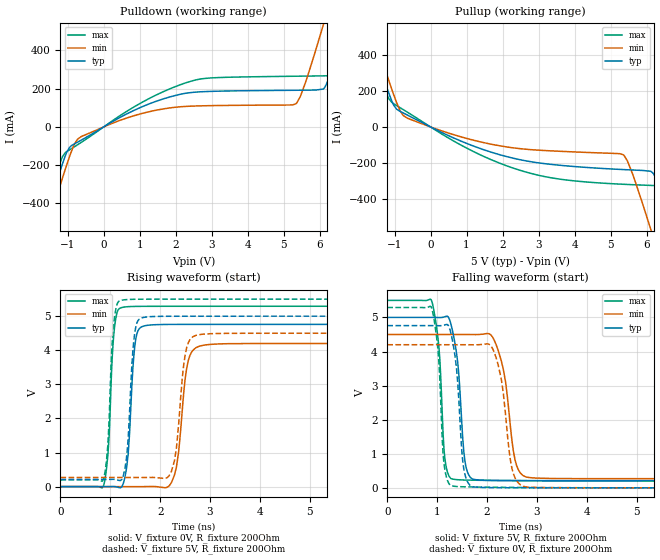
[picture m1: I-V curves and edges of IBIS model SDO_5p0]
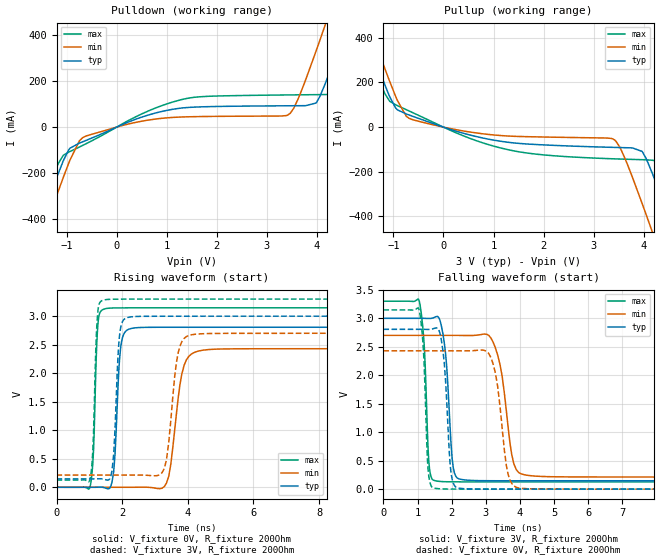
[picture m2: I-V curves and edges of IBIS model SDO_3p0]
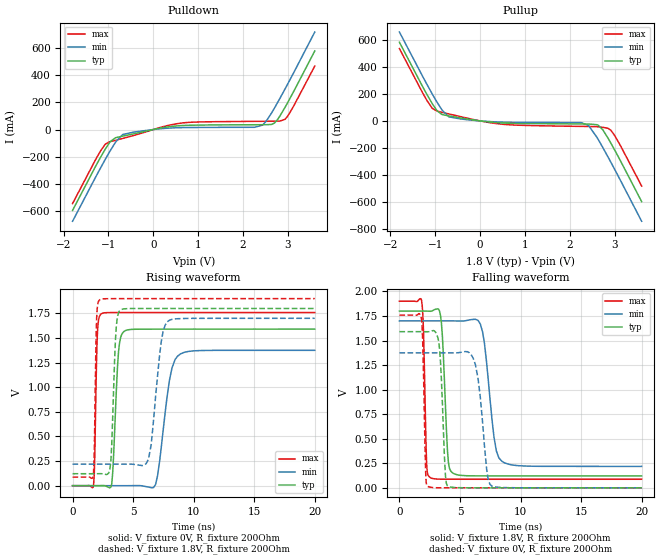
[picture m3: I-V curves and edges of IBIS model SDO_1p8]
|Texas Instruments Incorporated
|Quad, True 14-Bit, SPI Voltage-Output DAC With Precision Internal Reference
[IBIS Ver]   4.1
[File name]   dacx0504.ibs
[File Rev]   1.0
[Date]   01/27/2017
[Source]
| Texas Instruments Incorporated.
| 12500 TI Blvd
| Dallas, TX -75243
[Notes]   Revision History:
| Rev 1.0: 01/27/2017
| - Initial version of the model
| - Model generated from simulations in TISPICE
| - C_comp although listed in numerical order of value are
|   obtained from varying PVT conditions. For PVT conditions for
|   each specific value refer the buffer description under
|   respective [Model]. IBIS model user is responsible for using
|   appropriate C_comp to simulate for Signal Integrity.
| - Warnings regarding combined Non-monotonicity of various models have been
|   reviewd and considered minor and can be ignored.
| - Model names with a trailing _1p8 contain the model for
|   1.8V operation. Model names with a trailing _3p0 contain the model
|   for 3.3V operation.Model names with a trailing _5p0 contain the model
|   for 5.0V operation.
[Disclaimer]
| This model is designed as an aid for customers of Texas Instruments.
| TI and its licensors and suppliers make no warranties, either expressed
| or implied, with respect to this  model, including the warranties of
| merchantability or fitness for a particular purpose. The model is
| provided solely on an "as is" basis. The entire risk as to its quality
| and performance is with the customer.
[Copyright]
 (C) Copyright 2017 Texas Instruments Incorporated.All rights reserved.
|   Device
[Component]  DAC70504RTE
[Manufacturer]   TI
[Package]  |16 pin WQFN
| variable   typ   min   max
R_pkg   0.1   0.08   0.12
L_pkg   1.0nH   0.8nH   1.2nH
C_pkg   0.2pF   0.16pF   0.24pF
[Pin]   signal_name   model_name   R_pin   L_pin   C_pin
1   REF   NC   NA   NA   NA
2   OUT0   NC   NA   NA   NA
3   OUT1   NC   NA   NA   NA
4   OUT2   NC   NA   NA   NA
5   OUT3   NC   NA   NA   NA
6   GND   GND   NA   NA   NA
7   VDD   POWER   NA   NA   NA
8   GAIN   SDI   NA   NA   NA
9   RSTSEL   SDI   NA   NA   NA
10   REFDIV   SDI   NA   NA   NA
11   LDACB   SDI   NA   NA   NA
12   CSB   SDI   NA   NA   NA
13   SCLK   SDI   NA   NA   NA
14   SDI   SDI   NA   NA   NA
15   SDO/ALARMB   SDO   NA   NA   NA
16   VIO   POWER   NA   NA   NA
|   Model Selectors
[Model Selector]  SDO
SDO_5p0  sdata buffer at 5.0V operation.
SDO_3p0  sdata buffer at 3.0V operation.
SDO_1p8  sdata buffer at 1.8V operation.
[Model Selector]  SDI
SDI_5p0  sdata buffer at 5.0V operation.
SDI_3p0  sdata buffer at 3.0V operation.
SDI_1p8  sdata buffer at 1.8V operation.
| Models and submodels in the file (6): SDO_5p0 (Output), SDO_3p0 (Output), SDO_1p8 (Output), SDI_5p0 (Input), SDI_3p0 (Input), SDI_1p8 (Input)
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|   Model
[Model]   SDO_5p0
Model_type   Output
Polarity   Non-Inverting
Vmeas = 2.5
Vref = 0
Cref = 1pF
Rref = 100000
|   typ   min   max
C_comp   1pF   1pF   1pF
[Voltage Range]   5   4.5   5.5
[Temperature Range]   27   125   -40
[Pullup Reference]   5   4.5   5.5
[Pulldown Reference]   0   0   0
[Power Clamp Reference]   5   4.5   5.5
[GND Clamp Reference]   0   0   0
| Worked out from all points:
|   slope of the pulldown table from 0 to 0.75 V, typ, clamps not added: 9.61 ohm
|   slope of the pullup table from 0 to 0.75 V, typ, clamps not added: 10.7 ohm
|   falling waveform, V_fixture 5V, R_fixture 200Ohm: 20-80 % time 149ps typ, 227ps min, 119ps max; typ from 5 V to 0.211 V
|   rising waveform, V_fixture 0V, R_fixture 200Ohm: 20-80 % time 112ps typ, 167ps min, 100ps max; typ from 0 V to 4.76 V
|   rising waveform, V_fixture 5V, R_fixture 200Ohm: 20-80 % time 111ps typ, 156ps min, 96.4ps max; typ from 0.211 V to 5 V
|   falling waveform, V_fixture 0V, R_fixture 200Ohm: 20-80 % time 139ps typ, 206ps min, 114ps max; typ from 4.76 V to 0 V
[Pulldown]
|   Voltage   I(typ)   I(min)   I(max)
-5V       -2.704A    -2.779A    -2.658A
-2.195V   -855.7mA   -935.1mA   -805.9mA
-1.58V    -458.8mA   -539.1mA   -408.2mA
-1.145V   -193.2mA   -268.4mA   -155.8mA
-725mV    -79.65mA   -64.21mA   -93.36mA
640mV     67.98mA    46.69mA    81.52mA
2.65V     183.4mA    110.1mA    249.6mA
5.335V    191.9mA    120.8mA    265.3mA
6.1V      198.3mA    533.1mA    267.3mA
6.805V    589.9mA    986.3mA    275.3mA
7.27V     890.2mA    1.289A     522.8mA
10V       2.688A     3.088A     2.314A
[Pullup]
|   Voltage   I(typ)   I(min)   I(max)
-5V       2.688A     2.757A     2.645A
-2.15V    810.1mA    884.5mA    764mA
-1.73V    538.5mA    613.7mA    491.9mA
-1.655V   490.6mA    565.7mA    443.9mA
-1.16V    187.2mA    257.5mA    156mA
-755mV    76.9mA     62.84mA    95.4mA
2.245V    -170.6mA   -114.3mA   -224.3mA
5.35V     -235.8mA   -153.8mA   -317.2mA
6.1V      -245mA     -555.8mA   -323.4mA
6.865V    -646.4mA   -1.048A    -338.7mA
7.3V      -927.2mA   -1.331A    -557.5mA
10V       -2.705A    -3.11A     -2.328A
[Ramp]
R_load = 200
|   typ   min   max
dV/dt_r   2.85629/1.11775e-10   2.51978/1.67498e-10   3.17481/1.00389e-10
dV/dt_f   2.87354/1.49374e-10   2.53929/2.27194e-10   3.18142/1.19398e-10
[Falling Waveform]
V_fixture = 5V
V_fixture_min = 4.5V
V_fixture_max = 5.5V
R_fixture = 200Ohm
C_fixture = 0F
|   Time   V(typ)   V(min)   V(max)
0s        5V         4.5V       5.5V
880.1ps   5V         4.5V       5.521V
1.037ns   4.997V     4.5V       4.086V
1.153ns   5.02V      4.5V       881.8mV
1.317ns   4.547V     4.5V       255.7mV
1.555ns   801.4mV    4.5V       229.4mV
1.767ns   241.5mV    4.497V     224.1mV
2.181ns   217mV      4.205V     215.8mV
2.852ns   213.6mV    301.8mV    207.9mV
20ns      210.7mV    267.8mV    197.6mV
[Rising Waveform]
V_fixture = 0V
V_fixture_min = 0V
V_fixture_max = 0V
R_fixture = 200Ohm
C_fixture = 0F
|   Time   V(typ)   V(min)   V(max)
0s        19.62uV    26.57uV    14.41uV
861.1ps   -180.9uV   -40.74uV   7.327mV
1.087ns   861.4uV    -58.37uV   4.697V
1.275ns   167.7mV    -73.07uV   5.267V
1.511ns   4.328V     -91.53uV   5.286V
1.712ns   4.724V     1.13mV     5.288V
2.225ns   4.758V     113.5mV    5.291V
2.562ns   4.759V     3.688V     5.291V
2.929ns   4.759V     4.16V      5.291V
20ns      4.761V     4.2V       5.291V
[Rising Waveform]
V_fixture = 5V
V_fixture_min = 4.5V
V_fixture_max = 5.5V
R_fixture = 200Ohm
C_fixture = 0F
|   Time   V(typ)   V(min)   V(max)
0s        210.7mV    267.8mV    197.6mV
861.1ps   210.6mV    267.8mV    206.8mV
1.069ns   213.7mV    267.8mV    4.778V
1.236ns   229.2mV    267.8mV    5.471V
1.49ns    4.509V     267.8mV    5.496V
1.666ns   4.963V     268mV      5.498V
2.225ns   4.997V     442.6mV    5.499V
2.502ns   4.999V     3.87V      5.499V
2.783ns   4.999V     4.458V     5.499V
20ns      5V         4.5V       5.5V
[Falling Waveform]
|Gnd
V_fixture = 0V
V_fixture_min = 0V
V_fixture_max = 0V
R_fixture = 200Ohm
C_fixture = 0F
|   Time   V(typ)   V(min)   V(max)
0s        4.761V     4.2V       5.291V
880.1ps   4.761V     4.2V       5.311V
1.137ns   4.775V     4.2V       709.1mV
1.317ns   4.241V     4.2V       52.06mV
1.533ns   562.4mV    4.2V       31.34mV
1.712ns   31.19mV    4.198V     25.67mV
2.143ns   5.842mV    3.982V     17.63mV
2.502ns   2.991mV    560mV      13.5mV
2.783ns   2.259mV    25.26mV    10.82mV
20ns      19.87uV    27.03uV    14.9uV
|   Model
[Model]   SDO_3p0
Model_type   Output
Polarity   Non-Inverting
Vmeas = 1.5
Vref = 0
Cref = 1pF
Rref = 100000
|   typ   min   max
C_comp   1pF   1pF   1pF
[Voltage Range]   3   2.7   3.3
[Temperature Range]   27   125   -40
[Pullup Reference]   3   2.7   3.3
[Pulldown Reference]   0   0   0
[Power Clamp Reference]   3   2.7   3.3
[GND Clamp Reference]   0   0   0
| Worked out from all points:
|   slope of the pulldown table from 0 to 0.45 V, typ, clamps not added: 11.3 ohm
|   slope of the pullup table from 0 to 0.45 V, typ, clamps not added: 14.7 ohm
|   falling waveform, V_fixture 3V, R_fixture 200Ohm: 20-80 % time 179ps typ, 323ps min, 126ps max; typ from 3 V to 0.147 V
|   rising waveform, V_fixture 0V, R_fixture 200Ohm: 20-80 % time 141ps typ, 306ps min, 101ps max; typ from 0 V to 2.81 V
|   rising waveform, V_fixture 3V, R_fixture 200Ohm: 20-80 % time 133ps typ, 256ps min, 99.8ps max; typ from 0.147 V to 3 V
|   falling waveform, V_fixture 0V, R_fixture 200Ohm: 20-80 % time 162ps typ, 279ps min, 119ps max; typ from 2.81 V to 0 V
[Pulldown]
|   Voltage   I(typ)   I(min)   I(max)
-3V       -1.383A    -1.461A    -1.334A
-1.74V    -560.3mA   -640.6mA   -509.8mA
-1.29V    -276.3mA   -355.7mA   -227.6mA
-1.065V   -146.5mA   -219.1mA   -122.6mA
-606mV    -57.46mA   -38.41mA   -71.8mA
1.329V    83.93mA    44.43mA    121.6mA
3.417V    93.05mA    52.27mA    140.3mA
3.984V    105.1mA    331.4mA    141.5mA
4.173V    192.7mA    449.4mA    142mA
4.65V     486.8mA    754.4mA    254mA
4.902V    648.8mA    917.7mA    410mA
6V        1.366A     1.636A     1.124A
[Pullup]
|   Voltage   I(typ)   I(min)   I(max)
-3V       1.366A     1.439A     1.322A
-1.749V   549.7mA    625mA      503mA
-1.074V   136mA      204.5mA    115.8mA
-615mV    48.56mA    33.25mA    64.91mA
1.275V    -67.36mA   -39.59mA   -100.3mA
3.381V    -90.56mA   -52.6mA    -141.7mA
3.966V    -108.5mA   -340.8mA   -145.8mA
4.173V    -207.5mA   -470.3mA   -148.4mA
4.506V    -411.3mA   -683mA     -188.9mA
4.767V    -577.9mA   -851.6mA   -338.2mA
4.893V    -659.2mA   -933.3mA   -417.3mA
6V        -1.383A    -1.658A    -1.137A
[Ramp]
R_load = 200
|   typ   min   max
dV/dt_r   1.68391/1.41258e-10   1.45763/3.05913e-10   1.88848/1.00573e-10
dV/dt_f   1.71187/1.78517e-10   1.49191/3.23449e-10   1.90378/1.2617e-10
[Falling Waveform]
V_fixture = 3V
V_fixture_min = 2.7V
V_fixture_max = 3.3V
R_fixture = 200Ohm
C_fixture = 0F
|   Time   V(typ)   V(min)   V(max)
0s        3V         2.7V       3.3V
1.05ns    3V         2.7V       3.307V
1.192ns   2.999V     2.7V       2.559V
1.328ns   2.997V     2.7V       501.8mV
1.526ns   3.025V     2.7V       147.3mV
2.046ns   381.1mV    2.7V       129.5mV
2.257ns   174.5mV    2.699V     128.4mV
3.213ns   148mV      2.583V     127.7mV
4.12ns    147.6mV    254.1mV    127.6mV
20ns      146.9mV    213.5mV    127mV
[Rising Waveform]
V_fixture = 0V
V_fixture_min = 0V
V_fixture_max = 0V
R_fixture = 200Ohm
C_fixture = 0F
|   Time   V(typ)   V(min)   V(max)
0s        14.5uV     22.32uV    10.14uV
1.025ns   -63.32uV   -17.54uV   13.71mV
1.266ns   1.454mV    -26.94uV   2.893V
1.461ns   -8.28mV    -34.49uV   3.127V
1.985ns   2.561V     -54.88uV   3.145V
2.257ns   2.781V     -65.46uV   3.146V
3.347ns   2.806V     68.51mV    3.147V
3.82ns    2.806V     1.988V     3.147V
4.316ns   2.806V     2.387V     3.147V
20ns      2.807V     2.429V     3.147V
[Rising Waveform]
V_fixture = 3V
V_fixture_min = 2.7V
V_fixture_max = 3.3V
R_fixture = 200Ohm
C_fixture = 0F
|   Time   V(typ)   V(min)   V(max)
0s        146.9mV    213.5mV    127mV
1.025ns   146.8mV    213.7mV    148.3mV
1.246ns   147.8mV    213.8mV    2.993V
1.423ns   142.8mV    213.8mV    3.28V
1.69ns    290.3mV    213.9mV    3.297V
1.904ns   2.562V     213.9mV    3.298V
2.156ns   2.975V     214mV      3.299V
3.28ns    2.999V     323.3mV    3.299V
4.12ns    3V         2.675V     3.299V
20ns      3V         2.7V       3.3V
[Falling Waveform]
|Gnd
V_fixture = 0V
V_fixture_min = 0V
V_fixture_max = 0V
R_fixture = 200Ohm
C_fixture = 0F
|   Time   V(typ)   V(min)   V(max)
0s        2.807V     2.429V     3.147V
1.05ns    2.807V     2.429V     3.144V
1.308ns   2.805V     2.429V     355mV
1.461ns   2.818V     2.429V     22.2mV
1.742ns   2.442V     2.429V     4.153mV
1.957ns   423.2mV    2.429V     1.894mV
2.156ns   23.51mV    2.429V     1.304mV
3.15ns    878.1uV    2.309V     607uV
3.96ns    836.6uV    20.08mV    578.3uV
20ns      14.51uV    22.62uV    10.45uV
|   Model
[Model]   SDO_1p8
Model_type   Output
Polarity   Non-Inverting
Vmeas = 0.9
Vref = 0
Cref = 1pF
Rref = 100000
|   typ   min   max
C_comp   1pF   1pF   1pF
[Voltage Range]   1.8   1.7   1.9
[Temperature Range]   27   125   -40
[Pullup Reference]   1.8   1.7   1.9
[Pulldown Reference]   0   0   0
[Power Clamp Reference]   1.8   1.7   1.9
[GND Clamp Reference]   0   0   0
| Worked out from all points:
|   slope of the pulldown table from 0 to 0.27 V, typ, clamps not added: 16 ohm
|   slope of the pullup table from 0 to 0.27 V, typ, clamps not added: 27.5 ohm
|   falling waveform, V_fixture 1.8V, R_fixture 200Ohm: 20-80 % time 354ps typ, 729ps min, 196ps max; typ from 1.8 V to 0.122 V
|   rising waveform, V_fixture 0V, R_fixture 200Ohm: 20-80 % time 354ps typ, 835ps min, 170ps max; typ from 0 V to 1.59 V
|   rising waveform, V_fixture 1.8V, R_fixture 200Ohm: 20-80 % time 290ps typ, 695ps min, 142ps max; typ from 0.122 V to 1.8 V
|   falling waveform, V_fixture 0V, R_fixture 200Ohm: 20-80 % time 322ps typ, 631ps min, 184ps max; typ from 1.59 V to 0 V
[Pulldown]
|   Voltage   I(typ)   I(min)   I(max)
-1.8V     -598.2mA   -678.6mA   -547.7mA
-1.292V   -275.9mA   -356.1mA   -226.2mA
-1.076V   -148mA     -224.2mA   -111.2mA
-957.6mV  -89.38mA   -155.2mA   -89.16mA
-682.2mV  -49mA      -36.78mA   -65.97mA
651.6mV   29.67mA    14.25mA    48.73mA
2.261V    35.45mA    16.64mA    60.5mA
2.439V    35.66mA    33.11mA    60.91mA
2.704V    48.95mA    160mA      61.53mA
2.941V    166.7mA    302.6mA    77.33mA
3.13V     281.7mA    420.7mA    174.1mA
3.6V      581.1mA    721.1mA    469.6mA
[Pullup]
|   Voltage   I(typ)   I(min)   I(max)
-1.8V     581.7mA    657.2mA    534.8mA
-1.287V   256.2mA    331.9mA    209.8mA
-1.071V   129mA      200.8mA    94.66mA
-855mV    48.15mA    82.85mA    63.7mA
-698.4mV  36.92mA    30.17mA    51.56mA
516.6mV   -15.52mA   -9.275mA   -25.37mA
2.25V     -22.78mA   -12.99mA   -40.55mA
2.417V    -23.3mA    -34.6mA    -41.2mA
2.633V    -32.27mA   -138.4mA   -43.76mA
2.92V     -167.6mA   -309.4mA   -71.58mA
3.119V    -290mA     -434.6mA   -178.1mA
3.6V      -596.9mA   -742.4mA   -481.7mA
[Ramp]
R_load = 200
|   typ   min   max
dV/dt_r   0.95405/3.5442e-10   0.82486/8.34604e-10   1.05536/1.69955e-10
dV/dt_f   1.00705/3.53833e-10   0.888944/7.28623e-10   1.08761/1.96409e-10
[Falling Waveform]
V_fixture = 1.8V
V_fixture_min = 1.7V
V_fixture_max = 1.9V
R_fixture = 200Ohm
C_fixture = 0F
|   Time   V(typ)   V(min)   V(max)
0s        1.8V       1.7V       1.9V
1.833ns   1.8V       1.7V       1.905V
2.246ns   1.8V       1.7V       246mV
2.499ns   1.798V     1.7V       108.7mV
3.389ns   1.756V     1.7V       88.14mV
3.965ns   380.5mV    1.7V       87.58mV
4.321ns   158.9mV    1.7V       87.53mV
6.686ns   121.8mV    1.666V     87.35mV
8.47ns    121.6mV    269.3mV    87.34mV
20ns      121.6mV    218.4mV    87.3mV
[Rising Waveform]
V_fixture = 0V
V_fixture_min = 0V
V_fixture_max = 0V
R_fixture = 200Ohm
C_fixture = 0F
|   Time   V(typ)   V(min)   V(max)
0s        13.64uV    24.04uV    7.902uV
1.735ns   -46.57uV   -63.63nV   5.962mV
2.063ns   -57.96uV   -4.627uV   1.572V
2.378ns   965.6uV    -8.995uV   1.746V
3.234ns   17.07mV    -20.9uV    1.758V
3.8ns     1.364V     -28.76uV   1.759V
4.234ns   1.565V     -34.78uV   1.759V
6.857ns   1.59V      12.3mV     1.759V
8.941ns   1.59V      1.34V      1.759V
20ns      1.59V      1.375V     1.759V
[Rising Waveform]
V_fixture = 1.8V
V_fixture_min = 1.7V
V_fixture_max = 1.9V
R_fixture = 200Ohm
C_fixture = 0F
|   Time   V(typ)   V(min)   V(max)
0s        121.6mV    218.4mV    87.3mV
1.695ns   121.5mV    218.4mV    94.63mV
1.984ns   121.6mV    218.4mV    1.687V
2.246ns   121.9mV    218.4mV    1.888V
3.065ns   152.8mV    218.4mV    1.899V
3.618ns   1.628V     218.4mV    1.9V
3.965ns   1.785V     218.4mV    1.9V
6.277ns   1.8V       272.5mV    1.9V
7.808ns   1.8V       1.663V     1.9V
20ns      1.8V       1.7V       1.9V
[Falling Waveform]
|Gnd
V_fixture = 0V
V_fixture_min = 0V
V_fixture_max = 0V
R_fixture = 200Ohm
C_fixture = 0F
|   Time   V(typ)   V(min)   V(max)
0s        1.59V      1.375V     1.759V
1.792ns   1.59V      1.375V     1.738V
1.914ns   1.59V      1.375V     1.522V
2.158ns   1.59V      1.375V     185mV
2.332ns   1.589V     1.375V     15.22mV
3.234ns   1.495V     1.375V     747.7uV
3.965ns   19.14mV    1.375V     210.3uV
6.277ns   275.8uV    1.253V     56.53uV
7.653ns   99.64uV    15.4mV     51.64uV
20ns      13.67uV    24.43uV    7.768uV
